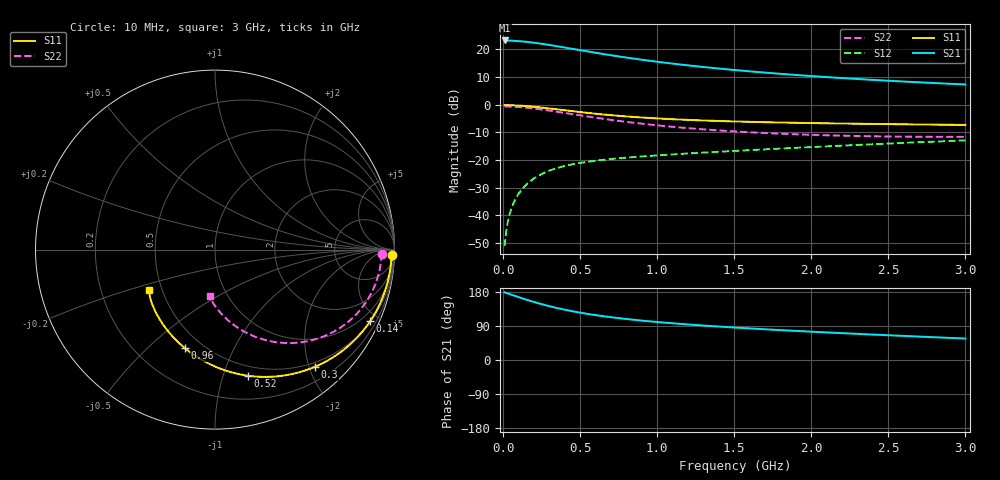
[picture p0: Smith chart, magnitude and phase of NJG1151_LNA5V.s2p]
! Created Fri Aug 03 14:55:36 2012
# hz S ma R 50
! 2 Port Network Data LNA section Port1:LNAIN  Port2:LNAOUT  VDD=5V,IDD=110mA  LNAIN connect GND Resistor(56kohm)
! freq  magS11  angS11  magS21  angS21  magS12  angS12  magS22  angS22
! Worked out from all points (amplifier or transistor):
!   300 points, 10 MHz to 3 GHz, reference 50 ohm
!   highest |S21| = 23.3 dB at 10 MHz (marker M1)
!   |S21| within 3 dB of that: start of sweep to 445 MHz
!   unconditionally stable (mu >= 1): nowhere
!   at 510 MHz: K = 0.31, MSG = 20.3 dB, |S12| = -21.0 dB
!   at 1.51 GHz: K = 0.69, MSG = 14.6 dB, |S12| = -16.7 dB
!   at 3 GHz: K = 0.87, MSG = 10.1 dB, |S12| = -12.9 dB
!   lowest NFmin = 0.19 dB at 10 MHz
!   S11 on the Smith chart (normalised r, x): 10 MHz: 25, -51; 140 MHz: 0.53, -4.50; 300 MHz: 0.42, -2.10; 520 MHz: 0.41, -1.21; 960 MHz: 0.40, -0.66; 3 GHz: 0.42, -0.24
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1e7  0.9845 -1.8  14.58 178.5  0.002761 61.6  0.9285 -1.4
3e7  0.9831 -5.4  14.53 175.7  0.007453 77.6  0.9271 -4.1
5e7  0.9805 -9.0  14.46 172.9  0.01229 79.7  0.9241 -6.8
9e7  0.9712 -16.1  14.26 167.3  0.02193 78.8  0.9137 -12.2
1.4e8  0.9522 -24.7  13.87 160.7  0.03352 75.4  0.8923 -18.8
1.8e8  0.9321 -31.4  13.49 155.6  0.0422 72.4  0.8696 -23.9
2.2e8  0.909 -37.8  13.04 150.8  0.05022 69.4  0.8434 -28.6
2.6e8  0.8839 -43.8  12.57 146.2  0.05753 66.6  0.8149 -33.1
3e8  0.858 -49.6  12.07 142.0  0.06415 64.0  0.7852 -37.3
3.9e8  0.8003 -61.2  10.96 133.5  0.07675 59.1  0.7181 -45.6
5.1e8  0.7314 -74.4  9.606 124.2  0.08962 54.4  0.6361 -54.7
5.2e8  0.7262 -75.4  9.501 123.5  0.09054 54.1  0.6299 -55.3
6.2e8  0.6792 -84.4  8.538 117.3  0.09874 51.4  0.5721 -61.4
7.2e8  0.6405 -92.2  7.714 111.9  0.1056 49.6  0.5232 -66.4
8.3e8  0.6061 -99.6  6.95 106.8  0.1122 48.3  0.4784 -71.1
9.6e8  0.574 -107.0  6.204 101.7  0.1193 47.4  0.4354 -75.7
1.01e9  0.5637 -109.5  5.955 99.9  0.1219 47.2  0.4213 -77.2
1.23e9  0.528 -118.9  5.053 92.9  0.1328 46.7  0.3712 -82.9
1.51e9  0.4979 -127.8  4.232 85.5  0.1466 46.8  0.3283 -88.1
2.01e9  0.4657 -138.3  3.291 74.5  0.1721 47.1  0.2851 -93.7
2.51e9  0.4457 -144.7  2.711 65.1  0.1991 46.8  0.2662 -95.9
3e9  0.4314 -148.2  2.328 56.6  0.2266 45.7  0.2626 -95.8
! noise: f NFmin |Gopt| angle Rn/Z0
1e+07  0.1874  0.7598  0.5364  0.1575
3.4e+08  0.4441  0.5188  19.31  0.1582
6.7e+08  0.8021  0.3058  45.56  0.157
1e+09  1.165  0.2138  85.5  0.1551
1.33e+09  1.52  0.2229  123.5  0.1529
1.67e+09  1.873  0.2697  146.8  0.1512
2e+09  2.201  0.3149  160.1  0.151
2.33e+09  2.511  0.3516  169.3  0.1533
2.66e+09  2.803  0.3791  176.3  0.1589
3e+09  3.085  0.3986  -177.6  0.1692
